FUNCTION_BLOCK FB_GetProductByBarCode
VAR_INPUT
	
END_VAR
VAR_IN_OUT
	fbClient:FB_IotHttpClient;
END_VAR
VAR_OUTPUT
	bBusy:BOOL;
	bError:BOOL;
	
	
END_VAR
VAR
	fbRequest			: FB_IotHttpRequest;
	fbJson				: FB_JsonDomParser;
	nState				: UDINT;
	RisingEdge			: R_TRIG;
	
	
	sUri:STRING;
	fbJsonDomParser		:FB_JsonDomParser;
	jsonDoc			:SJsonValue;
	
	emptyProduct:ST_Product;
END_VAR

//HMI
VAR
	bSend:BOOL;
	sBarCode:STRING;
	bProductNotFound:BOOL;
	nStatusCode:UINT;
	product:ST_Product;
	
END_VAR

RisingEdge(CLK:= bSend);
CASE nState OF
	0:
		sUri:=CONCAT('/Product/barcode/',sBarCode);
		IF RisingEdge.Q AND sBarCode<>'' THEN
			nStatusCode:=0;
			product:=emptyProduct;
			IF fbRequest.SendRequest(sUri:=sUri, fbClient:=fbClient, eRequestType:=ETcIotHttpRequestType.HTTP_Get, 0, 0, 0) THEN				
				nState:= 10;
				bBusy:= TRUE;
				bError:= FALSE;
				bProductNotFound:=FALSE;
			END_IF
		END_IF
		
	10:
		IF NOT fbRequest.bBusy THEN
			bError:=TRUE;
			nStatusCode:=fbRequest.nStatusCode;
			IF NOT fbRequest.bError THEN
				bError:=FALSE;
				IF fbRequest.nStatusCode=404 THEN
					bProductNotFound:=TRUE;
					nState:=100;
				END_IF
				IF fbRequest.nStatusCode=200 THEN
					jsonDoc:=fbRequest.GetJsonDomContent(fbJsonDomParser);
					IF jsonDoc<>0 THEN
						product.Id:=fbJsonDomParser.GetInt(fbJsonDomParser.FindMember(jsonDoc,'id'));
						product.CreatDateTime:=fbJsonDomParser.GetDateTime(fbJsonDomParser.FindMember(jsonDoc,'creatDateTime'));
						product.BarCode:=fbJsonDomParser.GetString(fbJsonDomParser.FindMember(jsonDoc,'barCode'));
						product.FinalPressure:=fbJsonDomParser.GetDouble(fbJsonDomParser.FindMember(jsonDoc,'finalPressure'));
						product.FinalDisplacement:=fbJsonDomParser.GetDouble(fbJsonDomParser.FindMember(jsonDoc,'finalDisplacement'));
						product.IsQualified:=fbJsonDomParser.GetBool(fbJsonDomParser.FindMember(jsonDoc,'isQualified'));
						nState:=100;
					END_IF
				END_IF
			END_IF
		END_IF
	100:
		bBusy:=FALSE;
		nState:=0;
END_CASE

END_FUNCTION_BLOCK
